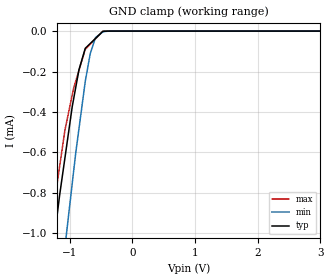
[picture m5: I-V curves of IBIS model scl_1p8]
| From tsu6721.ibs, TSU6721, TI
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|   scl_1p8 Model
[Model]   scl_1p8
Model_type   Input
Vinl = 0.54
Vinh = 1.26
|   typ   min   max
C_comp   1.124e-13   9.559e-14   1.141e-13
[Model spec]
|subparameter
Vinl   0.54   0.513   0.567
Vinh   1.26   1.197   1.323
[Voltage Range]   1.8   1.71   1.89
|Ambient Temperature   25   85   -40
|Junction Temperature
[Temperature Range]   27   125   -40
[Power Clamp Reference]   1.8   1.71   1.89
[GND Clamp Reference]   0   0   0
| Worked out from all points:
|   GND clamp passes 1 mA (typ) near -1.24 V on its own axis
[GND Clamp]
|   Voltage   I(typ)   I(min)   I(max)
-1.8V     -2.585mA   -3.51mA    -2.437mA
-1.329V   -1.228mA   -1.828mA   -1.052mA
-1.242V   -1.012mA   -1.561mA   -841.2uA
-1.075V   -624.9uA   -1.066mA   -488.3uA
-961.2mV  -375.8uA   -756.7uA   -317.7uA
-904.6mV  -279.3uA   -603.8uA   -248.1uA
-853.2mV  -192.1uA   -484uA     -194.9uA
-752.4mV  -85.38uA   -249.1uA   -90.43uA
-673.7mV  -61.77uA   -112.9uA   -65.24uA
-588.2mV  -36.11uA   -31.66uA   -37.99uA
-470.6mV  -1.091uA   -3.798uA   -515.8nA
3.6V      0A         0A         0A
[POWER Clamp]
|   Voltage   I(typ)   I(min)   I(max)
-1.8V     0A         0A         0A
0V        0A         0A         0A
3.6V      0A         0A         0A
